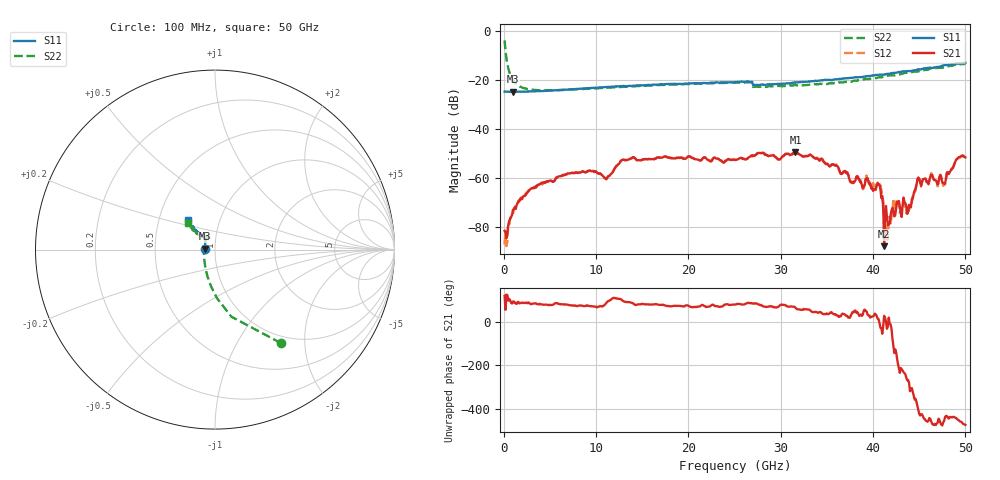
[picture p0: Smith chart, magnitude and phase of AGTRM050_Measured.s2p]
! Filename4Jim: AG16_W2_AGTRM050_1115_LRM_1BW_LRM.s2p
! Calibration: AG02 LRM + TRL
! Notes:
! Row:11, Col:15
! Probes: nan
! Prober: MPI TS150
! Date: 2023-09-21 15:18:55
! DC: None
# GHz S dB R 50
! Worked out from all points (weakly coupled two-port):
!   500 points, 100 MHz to 50 GHz, reference 50 ohm
!   highest |S21| = -49.37 dB at 31.6 GHz (marker M1); lowest = -87.8 dB at 41.2 GHz (marker M2)
!   lowest |S11| = -24.8 dB at 1 GHz (marker M3), VSWR 1.12, Z = 44.6 + j0.477 ohm
!   |S11| at or under -10 dB: start of sweep to end of sweep
!   |S22| runs from -24.3 to -3.9 dB; largest |S21 - S12| = 0.00024
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0.1  -24.79 179.3  -81.56 117.4  -87.11 130.8  -3.91 -54.8
0.4  -24.82 177.7  -82.14 120.4  -85.77 129.4  -13.59 -95.7
1  -24.85 174.7  -72.99 92.0  -74.53 89.0  -20.06 -124.7
3.8  -24.60 161.7  -62.87 78.7  -62.29 79.3  -24.22 -176.4
8.5  -23.53 144.7  -57.28 72.0  -57.25 71.7  -23.72 152.6
11.1  -22.95 137.9  -60.55 84.1  -60.41 85.5  -23.20 142.9
12.9  -22.49 134.1  -52.58 94.8  -52.59 94.7  -22.86 137.4
16.8  -21.91 130.4  -51.58 76.5  -51.68 77.6  -22.13 129.1
25.1  -20.93 130.0  -52.64 78.1  -52.73 78.7  -21.11 122.0
31.6  -21.07 125.6  -49.37 63.0  -49.37 63.8  -22.11 119.9
33.4  -20.51 127.4  -51.10 44.2  -51.02 43.9  -22.01 123.7
37.7  -19.15 131.6  -61.61 37.2  -61.63 33.4  -20.67 133.0
40.6  -17.95 134.2  -62.90 10.8  -62.91 13.3  -18.99 136.8
41.2  -17.78 134.7  -87.84 26.2  -75.21 2.3  -18.40 137.2
41.7  -17.57 135.1  -78.79 18.3  -76.05 7.1  -18.22 136.7
42.4  -17.11 134.9  -75.18 -126.9  -70.13 -136.0  -18.08 137.4
43.4  -16.59 134.9  -69.75 124.2  -71.55 120.5  -17.25 137.9
43.9  -16.39 134.7  -70.97 79.9  -72.86 77.6  -16.88 138.1
44.9  -15.76 135.4  -59.91 -44.2  -59.87 -45.1  -16.56 137.7
47.7  -13.97 134.5  -62.32 -94.0  -62.02 -93.7  -14.76 137.9
49.1  -13.44 131.3  -52.25 -86.2  -52.37 -81.6  -13.62 135.7
50  -12.99 132.8  -51.62 -112.8  -51.74 -111.9  -13.49 134.7
